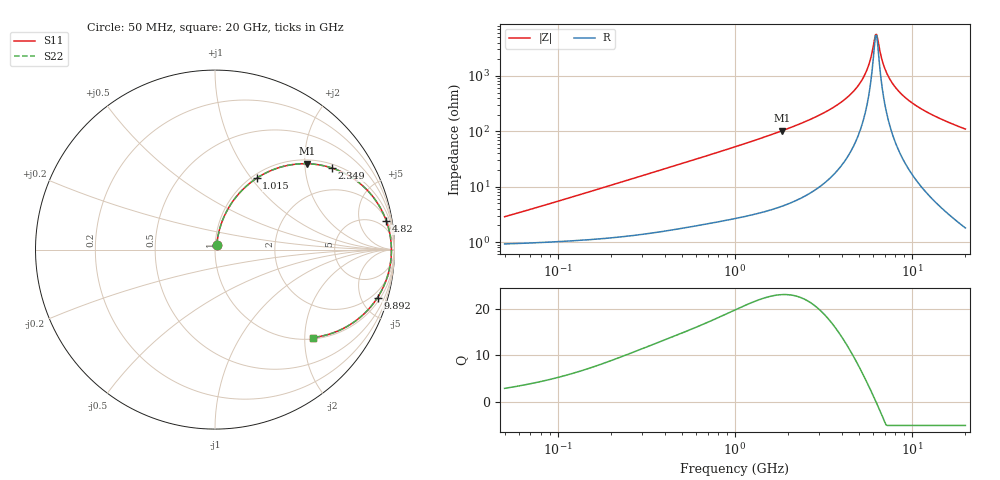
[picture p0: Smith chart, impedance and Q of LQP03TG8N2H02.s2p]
!Murata Part Number: LQP03TG8N2H02
!These Parameters are Measured in Series Mode Connection
!  o--[Z]--o
!Port1  Port2
!  o-------o
!Freq. Start=50[MHz] Stop=20[GHz], 401[Steps]
# Hz S RI R 50
!Freq.(Hz) S11(Real) S11(Imag) S21(Real) S21(Imag) S12(Real) S12(Imag) S22(Real) S22(Imag)
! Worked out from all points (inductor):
!   401 points, 50 MHz to 20 GHz, reference 50 ohm
!   read as one part in series: L = 8.62 nH near 51.52 MHz
!   highest Q = 23 at 1.848 GHz (marker M1), where L = 8.82 nH
!   self-resonance near 6.218 GHz
!   S11 on the Smith chart (normalised r, x): 50 MHz: 1.02, +0.05; 1.015 GHz: 1.05, +1.06; 2.349 GHz: 1.12, +2.76; 4.82 GHz: 2, +12; 9.892 GHz: 1.35, -6.66; 20 GHz: 1.04, -2.19
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5e7  0.0099 0.0267  0.9901 -0.0267  0.9901 -0.0267  0.0099 0.0267
1.364002e8  0.0158 0.0708  0.9842 -0.0708  0.9842 -0.0708  0.0158 0.0708
3.721004e8  0.05 0.1825  0.95 -0.1825  0.95 -0.1825  0.05 0.1825
6.380365e8  0.1139 0.2886  0.8861 -0.2886  0.8861 -0.2886  0.1139 0.2886
1e9  0.227 0.3943  0.773 -0.3943  0.773 -0.3943  0.227 0.3943
1.015091e9  0.2321 0.3977  0.7679 -0.3977  0.7679 -0.3977  0.2321 0.3977
1.848039e9  0.5116 0.4786  0.4884 -0.4786  0.4884 -0.4786  0.5116 0.4786
2.348516e9  0.6494 0.4553  0.3506 -0.4553  0.3506 -0.4553  0.6494 0.4553
2.728004e9  0.7329 0.4193  0.2671 -0.4193  0.2671 -0.4193  0.7329 0.4193
3.792786e9  0.8858 0.287  0.1142 -0.287  0.1142 -0.287  0.8858 0.287
4.81993e9  0.9553 0.1574  0.0447 -0.1574  0.0447 -0.1574  0.9553 0.1574
5.515528e9  0.9761 0.0776  0.0239 -0.0776  0.0239 -0.0776  0.9761 0.0776
5.769027e9  0.98 0.0504  0.02 -0.0504  0.02 -0.0504  0.98 0.0504
6.125241e9  0.9827 0.0138  0.0173 -0.0138  0.0173 -0.0138  0.9827 0.0138
6.217679e9  0.9829 0.00464  0.0171 -0.00464  0.0171 -0.00464  0.9829 0.00464
6.406762e9  0.9829 -0.0137  0.0171 0.0137  0.0171 0.0137  0.9829 -0.0137
6.905011e9  0.9798 -0.0595  0.0202 0.0595  0.0202 0.0595  0.9798 -0.0595
7.442007e9  0.9724 -0.1048  0.0276 0.1048  0.0276 0.1048  0.9724 -0.1048
8.389408e9  0.9517 -0.1757  0.0483 0.1757  0.0483 0.1757  0.9517 -0.1757
9.892087e9  0.9057 -0.2671  0.0943 0.2671  0.0943 0.2671  0.9057 -0.2671
1.354865e10  0.7686 -0.4078  0.2314 0.4078  0.2314 0.4078  0.7686 -0.4078
2e10  0.545 -0.4898  0.455 0.4898  0.455 0.4898  0.545 -0.4898
